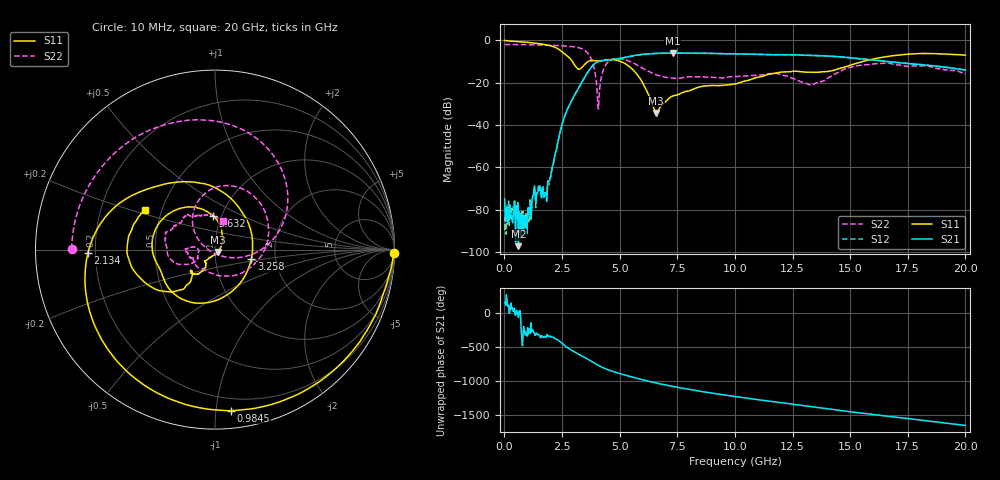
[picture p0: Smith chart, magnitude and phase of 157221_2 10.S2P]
!  2-Port S-parameters saved by WinCal
! VAR MeasName=S-Parameters (CALIBRATED_DATA) read from VNA (N5242A)
! VAR MeasDate=2015-5-26 16:47:50
! VAR NAME=157221_2 10
! VAR FILENAME=157221_2 10.S2P
! VAR DATE=2015-5-26 16:47:50
! VAR PHYS_PORTS=1,2
# Hz S DB R 50
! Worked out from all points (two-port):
!   801 points, 10 MHz to 20 GHz, reference 50 ohm
!   highest |S21| = -6.01 dB at 7.306 GHz (marker M1); lowest = -97.2 dB at 609.7 MHz (marker M2)
!   |S21| within 3 dB of the highest: 4.76 GHz to 15.73 GHz (10.97 GHz wide, 107 % of centre)
!   lowest |S11| = -34.3 dB at 6.582 GHz (marker M3), VSWR 1.04, Z = 51.4 - j1.31 ohm
!   |S11| at or under -10 dB: 2.952 GHz to 3.627 GHz (675.1 MHz wide, 20.5 % of centre); 5.053 GHz to 15.53 GHz (10.47 GHz wide, 102 % of centre)
!   |S22| runs from -32.4 to -2.0 dB; largest |S21 - S12| = 0.0094
!   S11 on the Smith chart (normalised r, x): 10 MHz: open; 984.5 MHz: 0.11, -1.10; 2.134 GHz: 0.17, -0.01; 3.258 GHz: 1.50, -0.17; 5.632 GHz: 0.91, +0.36; 20 GHz: 0.40, +0.22
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1e7  -0.03 -1.1  -74.77 159.9  -82.84 -118.1  -1.96 179.8
6.097e8  -0.58 -53.6  -97.20 -61.4  -90.96 8.7  -2.00 165.2
9.845125e8  -0.90 -84.3  -91.13 22.0  -84.62 24.3  -2.05 156.0
1.8091e9  -2.07 -149.8  -71.78 0.8  -71.00 3.8  -2.23 133.9
2.133938e9  -3.00 -178.5  -57.69 2.2  -57.91 0.3  -2.33 123.7
2.758625e9  -7.58 115.0  -32.04 -153.2  -32.02 -153.3  -2.71 99.4
3.258375e9  -13.56 -14.6  -21.68 107.9  -21.63 107.7  -3.54 70.6
3.358325e9  -12.82 -48.1  -19.76 90.0  -19.71 89.8  -3.93 62.7
3.783112e9  -9.49 -132.5  -12.53 9.4  -12.51 9.0  -9.11 13.0
4.082962e9  -9.77 -157.5  -9.94 -50.7  -9.94 -51.0  -32.44 -149.3
4.532738e9  -9.07 176.0  -9.27 -119.6  -9.26 -120.0  -9.87 99.1
5.632188e9  -14.53 93.0  -7.17 129.2  -7.17 128.8  -10.90 3.5
6.581712e9  -34.32 -41.5  -6.15 49.8  -6.16 49.6  -16.25 -71.7
6.681662e9  -33.08 -68.0  -6.13 42.3  -6.13 42.2  -16.51 -78.3
7.30635e9  -26.26 -117.9  -6.01 -0.8  -6.00 -1.1  -17.89 -109.3
8.630688e9  -21.61 -131.4  -6.07 -79.7  -6.07 -79.8  -17.29 -148.3
1.0005e10  -20.49 -121.7  -6.36 -150.0  -6.37 -150.4  -17.15 -160.1
1.192904e10  -15.06 -128.8  -6.76 122.1  -6.75 121.4  -15.86 178.1
1.335332e10  -15.02 -138.2  -7.14 58.6  -7.08 58.3  -20.85 -174.8
1.470265e10  -12.82 -127.2  -7.90 -1.5  -7.89 -1.8  -13.82 -155.9
1.667666e10  -7.51 -152.3  -10.07 -83.4  -10.06 -83.7  -10.82 160.3
2e10  -6.97 150.4  -13.96 142.6  -14.02 141.1  -15.75 74.7
